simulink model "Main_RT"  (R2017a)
settings: Solver=VariableStepAuto  StartTime=0.0  StopTime=50  FixedStep=1  RelTol=1e-3
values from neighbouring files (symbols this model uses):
  Hs_swlRange = zeros(states,N)    [run_master.m]
  Hsd_seaRange = zeros(states,N)    [run_master.m]
  Hsd_swlRange = zeros(states,N)    [run_master.m]
  m = 0    [wavespec.m]
  MC_Hs_swl = zeros(states,states,N)    [run_master.m]
  MC_Hsd_sea = zeros(states,states,N)    [run_master.m]
  MC_Hsd_swl = zeros(states,states,N)    [run_master.m]
  MC_Tp_sea = zeros(states,states,N)    [run_master.m]
  MC_Tp_swl = zeros(states,states,N)    [run_master.m]
  MC_u10 = zeros(states,states,N)    [run_master.m]
  MC_u10d = zeros(states,states,N)    [run_master.m]
  n = 0    [wavespec.m]
  Random_Values = generate_random_matrix(seed,SetNumRTs)    [run_master.m]    (also in generate_random_matrix.m = rand(Num_rand,8))
  Tp_seaRange = zeros(states,N)    [run_master.m]
  Tp_swlRange = zeros(states,N)    [run_master.m]
  u10_Range = zeros(states,N)    [run_master.m]
  u10d_Range = zeros(states,N)    [run_master.m]
  v_req_start = 14.5    [run_master.m]
  wpts = [32.8502 121.2880    [run_master.m]
undefined symbols (not defined in the file or in its folder): course_legs, course_legsBA, distnm_legs, distnm_legsBA, Hs_seaRange, MC_Hs_sea, ship_cargo_capacity

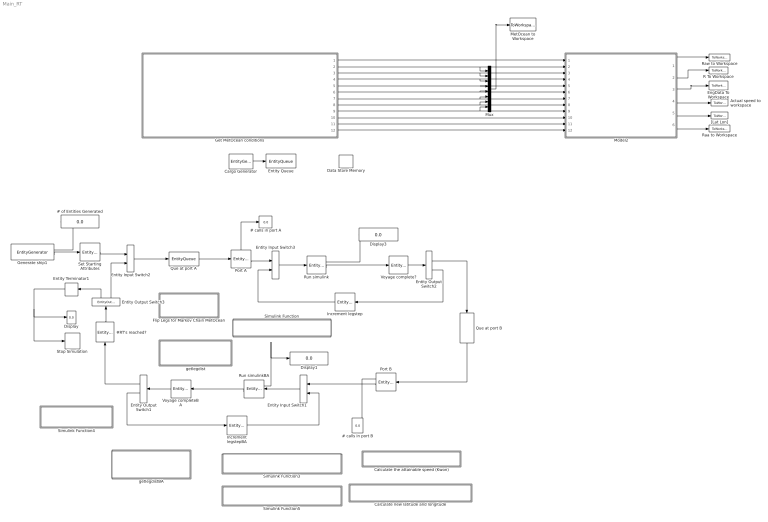
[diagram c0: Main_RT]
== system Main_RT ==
  # calls in port A : Display
  # calls in port B : Display
  # of Entities Generated : Display
  #RT's reached? : EntityServer  InputPortMessageModes=m  OutputPortMessageModes=m  Capacity=1  ServiceTimeValue=0  EntryAction=|
      | %Add to the number of round trips (RTs) completed
      | entity.NumRTs=entity.NumRTs+1;
      | 
      | %Check to see if the desired number of RTs is reached
      | %If so, send entity to terminate simulation
      | entity.outputport=Completed_RT(entity.NumRTs);
  Actual speed to workspace : ToWorkspace  VariableName=V_act  SaveFormat=Timeseries  SampleTime=-1
  Calculate new latitude and longitude : Subsystem  TreatAsAtomicUnit=on
  Calculate the attainable speed (Kwon) : Subsystem  TreatAsAtomicUnit=on
  Cargo Generator : EntityGenerator  Commented=on  OutputPortMessageModes=m  EntityType=Structured  EntityTypeName=Entity
  Data Store Memory : DataStoreMemory  ReadBeforeWriteMsg=warning  WriteAfterWriteMsg=warning  WriteAfterReadMsg=warning  ShowAdditionalParam=off
  Display : Display
  Display1 : Display
  Display3 : Display
  EngData To Workspace : ToWorkspace  VariableName=engroom  SaveFormat=Timeseries  SampleTime=-1
  Entity Input Switch1 : EntityInputSwitch  InputPortMessageModes=m,m  OutputPortMessageModes=m
  Entity Input Switch2 : EntityInputSwitch  InputPortMessageModes=m,m  OutputPortMessageModes=m
  Entity Input Switch3 : EntityInputSwitch  InputPortMessageModes=m,m  OutputPortMessageModes=m
  Entity Output Switch1 : EntityOutputSwitch  InputPortMessageModes=m  OutputPortMessageModes=m,m  SwitchingCriterion=From attribute  SwitchAttributeName=outputport
  Entity Output Switch2 : EntityOutputSwitch  InputPortMessageModes=m  OutputPortMessageModes=m,m  SwitchingCriterion=From attribute  SwitchAttributeName=outputport
  Entity Output Switch3 : EntityOutputSwitch  InputPortMessageModes=m  OutputPortMessageModes=m,m  SwitchingCriterion=From attribute  SwitchAttributeName=outputport
  Entity Queue : EntityQueue  Commented=on  InputPortMessageModes=m  OutputPortMessageModes=m
  Entity Terminator1 : EntityTerminator  InputPortMessageModes=m  NumberEntitiesArrived=on
  Flip Legs for Markov Chain MetOcean : Subsystem  TreatAsAtomicUnit=on
  Generate ship1 : EntityGenerator  OutputPortMessageModes=n,m  TimeSource=MATLAB action  IntergenerationTimeAction=|  GenerateEntityAtSimulationStart=off  AttributeName=HsSea_S|HsdSea_S|TpSea_S|HsSwl_S|HsdSwl_S|TpSwl_S|u10_S|u10d_S|speed|outputport|legstep|legdist|leg|course|lat|lon|Hs4k|Hsd4k|Att_speed|Dist_sailed_tot|Dist_sailed_leg|NumRTs|Voyage_step|capacity  AttributeInitialValue=0|0|0|0|0|0|0|0|15|1|2|1|1|1|1|1|1|1|1|0|0|0|0|1  NumberEntitiesDeparted=on  EntityType=Structured  EntityTypeName=ship
      | persistent count igt;
      | if isempty(count)
      |     igt=[0 inf];
      |     count=1;
      | end
      | dt=igt(count);
      | count=count+1;
  Get MetOcean conditions : Subsystem  TreatAsAtomicUnit=on
  Increment legstep : EntityServer  InputPortMessageModes=m  OutputPortMessageModes=m  Capacity=1  ServiceTimeValue=0  EntryAction=|
      | %increment the total progress
      | entity.legstep=entity.legstep+1;
  Increment legstepBA : EntityServer  InputPortMessageModes=m  OutputPortMessageModes=m  Capacity=1  ServiceTimeValue=0  EntryAction=|
      | %increment the total progress
      | entity.legstep=entity.legstep+1;
  MetOcean to Workspace : ToWorkspace  VariableName=MetOcean  SaveFormat=Timeseries  SampleTime=-1
  Model2 : ModelReference  ModelNameDialog=Ship_Model  SimulationMode=Normal  ModelReferenceVersion=1.112
  Mux : Mux  Inputs=8
  Port A : EntityServer  InputPortMessageModes=m  OutputPortMessageModes=n,m  Capacity=1  ServiceTimeValue=10  EntryAction=|  NumberEntitiesDeparted=on
      | %The ship is in port
      | 
      | %Run the ship model with the following modifications
      | %speed=0
      | %course=0
      | %Voyage_step: +0.5 (read as vessel being in port)
      | 
      | %run the ship model  and output the weather states (Markov Chain)
      | [HsSea_S,HsdSea_S,TpSea_S,HsSwl_S,HsdSwl_S,TpSwl_S,hsd4k,hs4k,u10_S,u10d_S]=runSim(entity.legstep, entity.course,entity.speed,entity.leg,...
      |                                                 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
  Port B : EntityServer  InputPortMessageModes=m  OutputPortMessageModes=n,m  Capacity=1  ServiceTimeValue=10  EntryAction=|  NumberEntitiesDeparted=on
      | %The ship is in port
      | 
      | %Run the ship model with the following modifications
      | %speed=0
      | %course=0
      | %Voyage_step: +0.5 (read as vessel being in port)
      | 
      | %run the ship model  and output the weather states (Markov Chain)
      | [HsSea_S,HsdSea_S,TpSea_S,HsSwl_S,HsdSwl_S,TpSwl_S,hsd4k,hs4k,u10_S,u10d_S]=runSim(entity.legstep, 0,0,entity.leg,...
      |                                                            entity.HsSwl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
  Que at port A : EntityQueue  InputPortMessageModes=m  OutputPortMessageModes=m
  Que at port B : EntityQueue  InputPortMessageModes=m  OutputPortMessageModes=m
  R To Workspace : ToWorkspace  VariableName=R  SaveFormat=Timeseries  SampleTime=-1
  Raa to Workspace : ToWorkspace  VariableName=Raa  SaveFormat=Timeseries  SampleTime=-1
  Raw to Workspace : ToWorkspace  VariableName=Raw  SaveFormat=Timeseries  SampleTime=-1
  Run simulink : EntityServer  InputPortMessageModes=m  OutputPortMessageModes=n,m  Capacity=1  ServiceTimeValue=1  EntryAction=|  NumberEntitiesDeparted=on
      | %take the current leg, and give the vessel its course and the distance of the leg
      | [entity.course,entity.legdist]=readLeg(entity.leg);
      | 
      | %run the ship model, and output the weather states (Markov Chain)
      | [HsSea_S,HsdSea_S,TpSea_S,HsSwl_S,HsdSwl_S,...
      |         TpSwl_S,hsd4k,hs4k,u10_S,u10d_S]  =  runSim(entity.legstep, entity.course,entity.speed,entity.leg,...
      |                                           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
  Run simulinkBA : EntityServer  InputPortMessageModes=m  OutputPortMessageModes=n,m  Capacity=1  ServiceTimeValue=1  EntryAction=|  NumberEntitiesDeparted=on
      | %take the current leg, and give the vessel its course and the distance of the leg
      | [entity.course,entity.legdist]=readLegBA(entity.leg); %reads from the flipped waypoints
      | 
      | %Flip leg number to collect the correct weather data for Markov Chain MetOcean
      | mc_leg=getmcleg(entity.leg);
      | 
      | %run the ship model, and output the weather states (Markov Chain)
      | [HsSea_S,HsdSea_S,TpSea_S,HsSwl_S,HsdSwl_S,...
      |        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
  Set Starting Attributes : EntityServer  InputPortMessageModes=m  OutputPortMessageModes=m  Capacity=1  ServiceTimeValue=0  EntryAction=|
      | %Read origin coordinates from waypoints
      | [lat1,lon1,v_req,capacity]=SetStart();
      | 
      | %Assign starting coordinates to entity
      | entity.lat=lat1;
      | entity.lon=lon1;
      | 
      | %Assign the intended speed
      | entity.speed=v_req;
      | 
      | %Assign cargo capacity
      | entity.capacity=capacity;
  Simulink Function : Subsystem  TreatAsAtomicUnit=on
  Simulink Function3 : Subsystem  TreatAsAtomicUnit=on
  Simulink Function4 : Subsystem  TreatAsAtomicUnit=on
  Simulink Function5 : Subsystem  TreatAsAtomicUnit=on
  Stop Simulation : Stop
  Voyage complete? : EntityServer  InputPortMessageModes=m  OutputPortMessageModes=m  Capacity=1  ServiceTimeValue=0  EntryAction=entity.outputport=checkComplete(entity.leg,entity.legdist,entity.Dist_sailed_leg);
  Voyage completeBA : EntityServer  InputPortMessageModes=m  OutputPortMessageModes=m  Capacity=1  ServiceTimeValue=0  EntryAction=entity.outputport=checkCompleteBA(entity.leg,entity.legdist,entity.Dist_sailed_leg);
  "[Lat Lon]" : ToWorkspace  VariableName=LatLon  SaveFormat=Timeseries  SampleTime=-1
  getlegdist : Subsystem  TreatAsAtomicUnit=on
  getlegdistBA : Subsystem  TreatAsAtomicUnit=on
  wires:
  Que at port B/1 -> Port B/1
  Entity Output Switch1/2 -> Increment legstepBA/1
  Port B/2 -> Entity Input Switch1/1
  Entity Input Switch1/1 -> Run simulinkBA/1
  Entity Input Switch2/1 -> Que at port A/1
  Cargo Generator/1 -> Entity Queue/1
  Model2/4 -> Actual speed to workspace/1
  Model2/2 -> R To Workspace/1
  Get MetOcean conditions/3(relD_sea) -> Model2/3, Mux/2
  Get MetOcean conditions/5(Hs_swl) -> Mux/4, Model2/5
  Get MetOcean conditions/2(Hs_sea) -> Mux/1, Model2/2
  Get MetOcean conditions/7(Tp_swl) -> Mux/6, Model2/7
  Get MetOcean conditions/1(vreq) -> Model2/1
  Model2/5 -> "[Lat Lon]"/1
  Model2/1 -> Raw to Workspace/1
  Get MetOcean conditions/6(relD_swl) -> Mux/5, Model2/6
  Get MetOcean conditions/4(Tp_sea) -> Mux/3, Model2/4
  Mux/1 -> MetOcean to Workspace/1
  Model2/3 -> EngData To Workspace/1
  Generate ship1/2 -> Set Starting Attributes/1
  Set Starting Attributes/1 -> Entity Input Switch2/1
  Generate ship1/1 -> # of Entities Generated/1
  Run simulinkBA/2 -> Voyage completeBA/1
  Voyage completeBA/1 -> Entity Output Switch1/1
  Increment legstepBA/1 -> Entity Input Switch1/2
  Run simulinkBA/1 -> Display1/1
  Port A/1 -> # calls in port A/1
  Port B/1 -> # calls in port B/1
  Entity Terminator1/1 -> Stop Simulation/1, Display/1
  Entity Output Switch3/2 -> Entity Input Switch2/2
  Entity Output Switch3/1 -> Entity Terminator1/1
  #RT's reached?/1 -> Entity Output Switch3/1
  Entity Output Switch1/1 -> #RT's reached?/1
  Entity Output Switch2/1 -> Que at port B/1
  Run simulink/1 -> Display3/1
  Entity Output Switch2/2 -> Increment legstep/1
  Voyage complete?/1 -> Entity Output Switch2/1
  Run simulink/2 -> Voyage complete?/1
  Increment legstep/1 -> Entity Input Switch3/2
  Entity Input Switch3/1 -> Run simulink/1
  Port A/2 -> Entity Input Switch3/1
  Que at port A/1 -> Port A/1
  Get MetOcean conditions/8(u10) -> Model2/8, Mux/7
  Get MetOcean conditions/9(relD_u10) -> Model2/9, Mux/8
  Get MetOcean conditions/10(Course) -> Model2/10
  Get MetOcean conditions/11(lat) -> Model2/11
  Get MetOcean conditions/12(lon) -> Model2/12
  Model2/6 -> Raa to Workspace/1

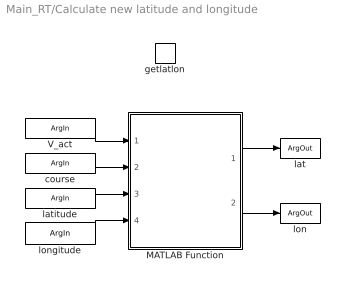
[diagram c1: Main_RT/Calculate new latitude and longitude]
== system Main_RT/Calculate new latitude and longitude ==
  getlatlon : TriggerPort  TriggerType=function-call  IsSimulinkFunction=on  FunctionName=getlatlon  VariantControl=Variant
  MATLAB Function : MATLAB Function  TreatAsAtomicUnit=on
  V_act : ArgIn  DisableCoverage=on  ArgumentName=V_act
  latitude : ArgIn  Port=2  ArgumentName=latitude
  longitude : ArgIn  Port=3  ArgumentName=longitude
  course : ArgIn  Port=4  ArgumentName=course
  lat : ArgOut  DisableCoverage=on  ArgumentName=lat
  lon : ArgOut  Port=2  ArgumentName=lon
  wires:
  V_act/1 -> MATLAB Function/1(V_act)
  MATLAB Function/1(lat_new) -> lat/1
  course/1 -> MATLAB Function/2(Course)
  latitude/1 -> MATLAB Function/3(Lat)
  longitude/1 -> MATLAB Function/4(Lon)
  MATLAB Function/2(lon_new) -> lon/1

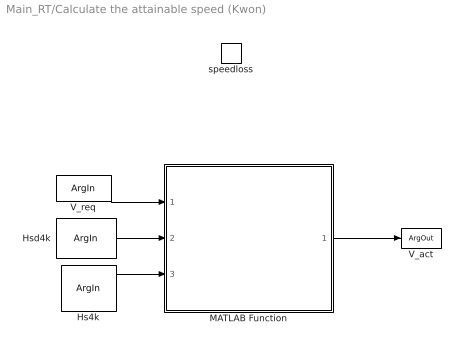
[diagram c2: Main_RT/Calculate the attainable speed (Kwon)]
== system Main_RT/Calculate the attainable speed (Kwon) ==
  speedloss : TriggerPort  TriggerType=function-call  IsSimulinkFunction=on  FunctionName=speedloss  VariantControl=Variant
  MATLAB Function : MATLAB Function  TreatAsAtomicUnit=on
  V_req : ArgIn  DisableCoverage=on  ArgumentName=V_req
  Hsd4k : ArgIn  Port=2  ArgumentName=Hsd4k
  Hs4k : ArgIn  Port=3  ArgumentName=Hs4k
  V_act : ArgOut  DisableCoverage=on  ArgumentName=V_act
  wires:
  MATLAB Function/1(V_act) -> V_act/1
  Hs4k/1 -> MATLAB Function/3(Hs)
  Hsd4k/1 -> MATLAB Function/2(rel_heading)
  V_req/1 -> MATLAB Function/1(V_req)

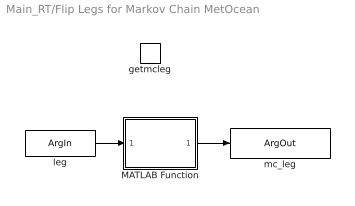
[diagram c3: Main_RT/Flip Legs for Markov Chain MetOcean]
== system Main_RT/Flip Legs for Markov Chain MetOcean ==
  getmcleg : TriggerPort  TriggerType=function-call  IsSimulinkFunction=on  FunctionName=getmcleg  VariantControl=Variant
  MATLAB Function : MATLAB Function  TreatAsAtomicUnit=on
  leg : ArgIn  DisableCoverage=on  ArgumentName=leg
  mc_leg : ArgOut  DisableCoverage=on  ArgumentName=mc_leg
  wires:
  leg/1 -> MATLAB Function/1(leg)
  MATLAB Function/1(mc_leg) -> mc_leg/1

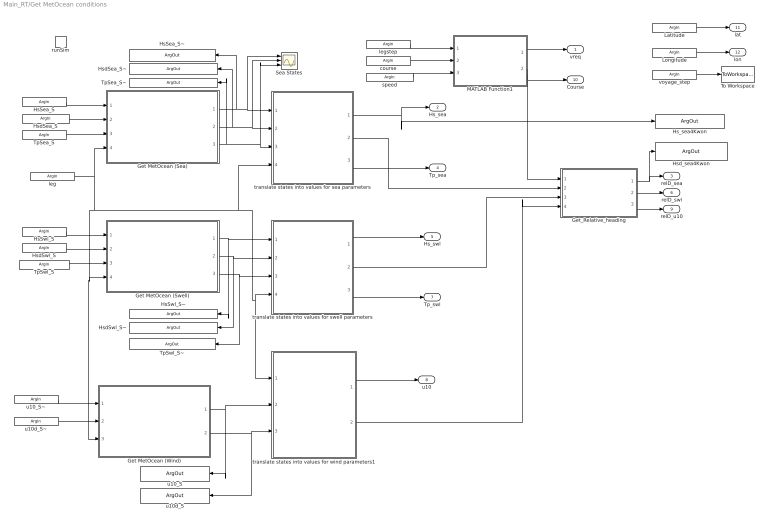
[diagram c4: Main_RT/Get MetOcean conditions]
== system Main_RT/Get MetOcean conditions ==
  runSim : TriggerPort  TriggerType=function-call  IsSimulinkFunction=on  FunctionName=runSim  VariantControl=Variant
  Get MetOcean (Sea) : MATLAB Function  TreatAsAtomicUnit=on
  Get MetOcean (Swell) : MATLAB Function  TreatAsAtomicUnit=on
  Get MetOcean (Wind) : MATLAB Function  TreatAsAtomicUnit=on
  Get_Relative_heading : MATLAB Function  TreatAsAtomicUnit=on
  MATLAB Function1 : MATLAB Function  TreatAsAtomicUnit=on
  Sea States : Scope  NumInputPorts=3
  To Workspace : ToWorkspace  VariableName=voyage_step  SaveFormat=Timeseries  SampleTime=-1
  translate states into values for swell parameters : MATLAB Function  TreatAsAtomicUnit=on
  translate states into values for wind parameters1 : MATLAB Function  TreatAsAtomicUnit=on
  translate states into values for sea parameters : MATLAB Function  TreatAsAtomicUnit=on
  legstep : ArgIn  ArgumentName=legstep
  course : ArgIn  Port=2  ArgumentName=course
  speed : ArgIn  Port=3  ArgumentName=speed
  leg : ArgIn  Port=4  ArgumentName=leg
  HsSwl_S : ArgIn  Port=5  ArgumentName=HsSwl_S
  HsdSwl_S : ArgIn  Port=6  ArgumentName=HsdSwl_S
  TpSwl_S : ArgIn  Port=7  ArgumentName=TpSwl_S
  HsSea_S : ArgIn  Port=8  ArgumentName=HsSea_S
  HsdSea_S : ArgIn  Port=9  ArgumentName=HsdSea_S
  TpSea_S : ArgIn  Port=10  ArgumentName=TpSea_S
  Latitude : ArgIn  Port=11  ArgumentName=Latitude
  Longitude : ArgIn  Port=12  ArgumentName=Longitude
  u10_S~ : ArgIn  Port=13  ArgumentName=u10_S
  u10d_S~ : ArgIn  Port=14  ArgumentName=u10d_S
  voyage_step : ArgIn  Port=15  ArgumentName=voyage_step
  HsSea_S~ : ArgOut  ArgumentName=HsSea_S
  HsdSea_S~ : ArgOut  Port=2  ArgumentName=HsdSea_S
  TpSea_S~ : ArgOut  Port=3  ArgumentName=TpSea_S
  HsSwl_S~ : ArgOut  Port=4  ArgumentName=HsSwl_S
  HsdSwl_S~ : ArgOut  Port=5  ArgumentName=HsdSwl_S
  TpSwl_S~ : ArgOut  Port=6  ArgumentName=TpSwl_S
  Hsd_sea4Kwon : ArgOut  Port=7  ArgumentName=Hsd_sea4Kwon
  Hs_sea4Kwon : ArgOut  Port=8  ArgumentName=Hs_sea4Kwon
  u10_S : ArgOut  Port=9  ArgumentName=u10_S
  u10d_S : ArgOut  Port=10  ArgumentName=u10d_S
  vreq : Outport
  Hs_sea : Outport  Port=2
  relD_sea : Outport  Port=3
  Tp_sea : Outport  Port=4
  Hs_swl : Outport  Port=5
  relD_swl : Outport  Port=6
  Tp_swl : Outport  Port=7
  u10 : Outport  Port=8
  relD_u10 : Outport  Port=9
  Course : Outport  Port=10
  lat : Outport  Port=11
  lon : Outport  Port=12
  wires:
  leg/1 -> Get MetOcean (Sea)/4(leg), Get MetOcean (Wind)/3(leg), Get MetOcean (Swell)/4(leg), translate states into values for wind parameters1/1(leg), translate states into values for swell parameters/4(leg), translate states into values for sea parameters/4(leg)
  Get MetOcean (Sea)/1(Sea_HSS) -> HsSea_S~/1, Sea States/1, translate states into values for sea parameters/1(HsSea_S)
  Get MetOcean (Sea)/2(Sea_HSDS) -> HsdSea_S~/1, Sea States/2, translate states into values for sea parameters/2(HsdSea_S)
  Get MetOcean (Sea)/3(Sea_TPS) -> TpSea_S~/1, Sea States/3, translate states into values for sea parameters/3(TpSea_S)
  translate states into values for sea parameters/1(Hs_sea) -> Hs_sea4Kwon/1, Hs_sea/1
  translate states into values for sea parameters/3(Tp_sea) -> Tp_sea/1
  Get MetOcean (Swell)/2(HSD_S) -> HsdSwl_S~/1, translate states into values for swell parameters/2(HsdSwl_S)
  Get MetOcean (Swell)/3(TM_S) -> TpSwl_S~/1, translate states into values for swell parameters/3(TpSwl_S)
  translate states into values for swell parameters/2(Hsd_swl) -> Get_Relative_heading/3(Hsd_swl)
  Get MetOcean (Swell)/1(HS_S) -> HsSwl_S~/1, translate states into values for swell parameters/1(HsSwl_S)
  translate states into values for swell parameters/1(Hs_swl) -> Hs_swl/1
  translate states into values for swell parameters/3(Tp_swl) -> Tp_swl/1
  MATLAB Function1/1(Vreq) -> vreq/1
  MATLAB Function1/2(Course) -> Get_Relative_heading/1(course), Course/1
  HsSea_S/1 -> Get MetOcean (Sea)/1(Hs_SeS)
  HsdSea_S/1 -> Get MetOcean (Sea)/2(Hsd_SeS)
  TpSea_S/1 -> Get MetOcean (Sea)/3(Tp_SeS)
  TpSwl_S/1 -> Get MetOcean (Swell)/3(Per_S)
  HsdSwl_S/1 -> Get MetOcean (Swell)/2(Head_S)
  HsSwl_S/1 -> Get MetOcean (Swell)/1(Wave_S)
  speed/1 -> MATLAB Function1/3(speed)
  course/1 -> MATLAB Function1/2(course)
  legstep/1 -> MATLAB Function1/1(legstep)
  Latitude/1 -> lat/1
  Longitude/1 -> lon/1
  u10_S~/1 -> Get MetOcean (Wind)/1(windVel_S)
  translate states into values for wind parameters1/1(u10) -> u10/1
  translate states into values for sea parameters/2(Hsd_sea) -> Get_Relative_heading/2(Hsd_sea)
  translate states into values for wind parameters1/2(u10d) -> Get_Relative_heading/4(u10d)
  Get_Relative_heading/3(relD_u10) -> relD_u10/1
  Get_Relative_heading/2(relD_swl) -> relD_swl/1
  Get_Relative_heading/1(relD_sea) -> Hsd_sea4Kwon/1, relD_sea/1
  Get MetOcean (Wind)/1(u10_S) -> u10_S/1, translate states into values for wind parameters1/2(u10_S)
  Get MetOcean (Wind)/2(u10d_S) -> u10d_S/1, translate states into values for wind parameters1/3(u10d_S)
  u10d_S~/1 -> Get MetOcean (Wind)/2(windDir_S)
  voyage_step/1 -> To Workspace/1

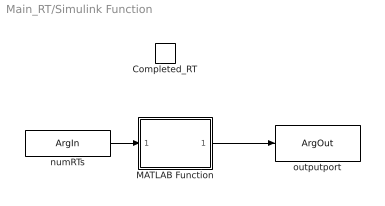
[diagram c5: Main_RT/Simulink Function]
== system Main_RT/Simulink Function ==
  Completed_RT : TriggerPort  TriggerType=function-call  IsSimulinkFunction=on  FunctionName=Completed_RT  VariantControl=Variant
  MATLAB Function : MATLAB Function  TreatAsAtomicUnit=on
  numRTs : ArgIn  DisableCoverage=on  ArgumentName=numRTs
  outputport : ArgOut  DisableCoverage=on  ArgumentName=outputport
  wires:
  numRTs/1 -> MATLAB Function/1(NumRTs)
  MATLAB Function/1(outport) -> outputport/1

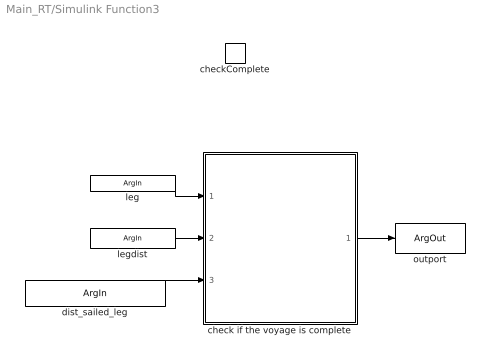
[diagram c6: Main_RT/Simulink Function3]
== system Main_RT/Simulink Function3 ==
  checkComplete : TriggerPort  TriggerType=function-call  IsSimulinkFunction=on  FunctionName=checkComplete  VariantControl=Variant
  check if the voyage is complete : MATLAB Function  TreatAsAtomicUnit=on
  leg : ArgIn  DisableCoverage=on  ArgumentName=leg
  legdist : ArgIn  Port=2  ArgumentName=legdist
  dist_sailed_leg : ArgIn  Port=3  ArgumentName=dist_sailed_leg
  outport : ArgOut  DisableCoverage=on  ArgumentName=outport
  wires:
  leg/1 -> check if the voyage is complete/1(leg)
  check if the voyage is complete/1(outport) -> outport/1
  dist_sailed_leg/1 -> check if the voyage is complete/3(dist_sailed_leg)
  legdist/1 -> check if the voyage is complete/2(legdist)

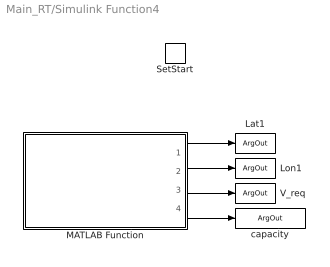
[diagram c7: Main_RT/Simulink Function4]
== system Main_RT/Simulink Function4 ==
  SetStart : TriggerPort  TriggerType=function-call  IsSimulinkFunction=on  FunctionName=SetStart  VariantControl=Variant
  MATLAB Function : MATLAB Function  TreatAsAtomicUnit=on
  Lat1 : ArgOut  DisableCoverage=on  ArgumentName=Lat1
  Lon1 : ArgOut  Port=2  ArgumentName=Lon1
  V_req : ArgOut  Port=3  ArgumentName=V_req
  capacity : ArgOut  Port=4  ArgumentName=capacity
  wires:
  MATLAB Function/2(Lon1) -> Lon1/1
  MATLAB Function/1(Lat1) -> Lat1/1
  MATLAB Function/3(v_req) -> V_req/1
  MATLAB Function/4(capacity) -> capacity/1

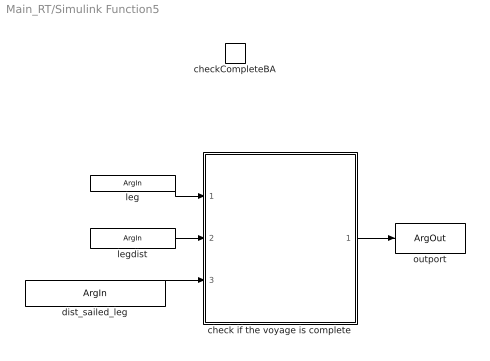
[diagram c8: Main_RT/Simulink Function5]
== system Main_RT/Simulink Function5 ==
  checkCompleteBA : TriggerPort  TriggerType=function-call  IsSimulinkFunction=on  FunctionName=checkCompleteBA  VariantControl=Variant
  check if the voyage is complete : MATLAB Function  TreatAsAtomicUnit=on
  leg : ArgIn  DisableCoverage=on  ArgumentName=leg
  legdist : ArgIn  Port=2  ArgumentName=legdist
  dist_sailed_leg : ArgIn  Port=3  ArgumentName=dist_sailed_leg
  outport : ArgOut  DisableCoverage=on  ArgumentName=outport
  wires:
  leg/1 -> check if the voyage is complete/1(leg)
  check if the voyage is complete/1(outport) -> outport/1
  dist_sailed_leg/1 -> check if the voyage is complete/3(dist_sailed_leg)
  legdist/1 -> check if the voyage is complete/2(legdist)

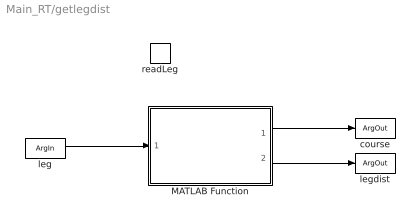
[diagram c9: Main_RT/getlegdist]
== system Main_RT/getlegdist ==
  readLeg : TriggerPort  TriggerType=function-call  IsSimulinkFunction=on  FunctionName=readLeg  VariantControl=Variant
  MATLAB Function : MATLAB Function  TreatAsAtomicUnit=on
  leg : ArgIn  DisableCoverage=on  ArgumentName=leg
  course : ArgOut  DisableCoverage=on  ArgumentName=course
  legdist : ArgOut  DisableCoverage=on  Port=2  ArgumentName=legdist
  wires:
  leg/1 -> MATLAB Function/1(leg)
  MATLAB Function/1(course) -> course/1
  MATLAB Function/2(legdist) -> legdist/1

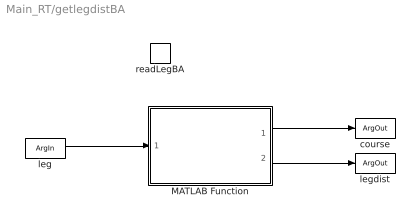
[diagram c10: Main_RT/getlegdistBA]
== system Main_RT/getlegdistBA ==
  readLegBA : TriggerPort  TriggerType=function-call  IsSimulinkFunction=on  FunctionName=readLegBA  VariantControl=Variant
  MATLAB Function : MATLAB Function  TreatAsAtomicUnit=on
  leg : ArgIn  DisableCoverage=on  ArgumentName=leg
  course : ArgOut  DisableCoverage=on  ArgumentName=course
  legdist : ArgOut  DisableCoverage=on  Port=2  ArgumentName=legdist
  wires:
  leg/1 -> MATLAB Function/1(leg)
  MATLAB Function/1(course) -> course/1
  MATLAB Function/2(legdist) -> legdist/1

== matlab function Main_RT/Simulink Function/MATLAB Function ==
function outport = outputportRT(NumRTs,SetNumRTs)



if NumRTs>=SetNumRTs
outport = 1; %Simulation is complete, end simulation
else
    outport=2; %Simulation is not complete, do another roundtrip
end
end

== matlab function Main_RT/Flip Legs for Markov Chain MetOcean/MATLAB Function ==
function mc_leg = getMCleg(leg,distnm_legsBA)

%Flip the leg number to collect the correct weather data for MetOcean
%Markov Chains

num_legs=size(distnm_legsBA,1); %get the total number of legs
legs=(1:1:num_legs);
flip_legs=flip(legs);
mc_leg=flip_legs(leg);
end

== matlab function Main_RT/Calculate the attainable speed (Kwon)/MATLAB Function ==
function V_act = speedloss_Kwon(V_req,rel_heading,Hs, num)
coder.extrinsic('wrapTo180')
%Use Kwons method to estimate the speed loss due to added resistance

%pre allocate values
V_act=0;
V_2=0; %pre allocate the new speed
Bn=0;
Volume_deplacement=0;
C_u=0;
C_beta=0;
C_form=0;
heading_rel=0;

V_1=V_req*0.5144; %Convert the required speed (set speed) from kts to m/s
heading_rel=abs(wrapTo180(rel_heading)); %convert to 0-180 degrees
Volume_deplacement=num(54); %[m^3]
L=num(3); %Use Lwl
C_B=num(8); %block Coefficient



%calculate the current Froude Number
F_n=V_1/((9.81*L)^0.5);

%Get Beaufort scale number from waveheight
if Hs<0.2
    Bn=1;
elseif Hs>=0.2 && Hs<0.5
    Bn=2;
elseif Hs>=0.5 && Hs<1
    Bn=3;
elseif Hs>=1 && Hs<2
    Bn=4;
elseif Hs>2 && Hs<3
    Bn=5;
elseif Hs>3 && Hs<4
    Bn=6;
elseif Hs>4 %&& Hs<5.5
    Bn=7;
else
    disp('Bn is too high for Kwons method')
end
    

%calculate speed reduction coefficient
if C_B>=0.55 && C_B<0.575
    C_u=1.7-(1.4*F_n)-(7.4*(F_n^2));
elseif C_B>=0.575 && C_B<0.625
    C_u=2.2-(2.5*F_n)-(9.7*(F_n^2));
elseif C_B>=0.625 && C_B<0.675
    C_u=2.6-(3.7*F_n)-(11.6*(F_n^2));
elseif C_B>=0.675 && C_B<0.725
    C_u=3.1-(5.3*F_n)-(12.4*(F_n^2));
elseif C_B>=0.725 && C_B<0.775
    C_u=2.4-(10.6*F_n)-(9.5*(F_n^2));
elseif C_B>=0.775 && C_B<0.825
    C_u=2.6-(13.1*F_n)-(15.1*(F_n^2));
else %C_B>=0.825
    C_u=3.1-(18.7*F_n)+(28*(F_n^2));
end

%calculate direction reduction coefficient
if heading_rel>=0 && heading_rel<30 %head sea
    C_beta=1;
elseif heading_rel>=30 && heading_rel<60 %Bow sea
    C_beta=(1.7-0.03*((Bn-4)^2))/2;
elseif heading_rel>=60 && heading_rel<150 %Beam sea
    C_beta=(0.9-0.06*((Bn-6)^2))/2;
else %heading_rel>=150 && heading_rel<180 %Following sea
    C_beta=(0.4-0.03*((Bn-8)^2))/2;
end

%calculate the ship form coefficient
%valid for all ships, exept container ships, in loaded condition
%C_form=(0.5*Bn)+((Bn^(6.5))/((2.7*(Volume_deplacement^(2/3)))));

%valid for container ships in normal condition
C_form=(0.7*Bn)+((Bn^(6.5))/((22*(Volume_deplacement^(2/3)))));

%percentage loss calculated
%percentage_loss=((V_1-V_2)/V_1)*100;





%calculate deltaV/V1*100%
%Delta_V_overV=C_beta*C_u*C_form;
%coefficient=C_form*C_beta*C_u
%calculate actual ship speed in the selected weather [m/s]
% V_2=V_1-((Delta_V_overV)*(V_1/100))
V_2=V_1-((C_beta*C_u*C_form)*(V_1/100));

%calculate the absolute speed loss [m/s]
%delta_V=V_1-V_2



%if the speed loss found is negative, set the speed to the original speed
% This means that the approximate method did not work in this case
% if V_2>=V_1
%     V_2=V_1; 
%     disp('Approximate method not valid')
%     
% end

V_act=V_2/0.5144; % The actual attainable speed in kts
end


% %function V_act = speedloss_Kwon(V_req,rel_heading,Hs, num)
% %Use Kwons method to estimate the speed loss due to added resistance
% 
% V_1=V_req*0.5144; %Convert the required speed (set speed) from kts to m/s
% heading_rel=rel_heading;
% Volume_deplacement=num(54); %[m^3]
% L=num(3); %Use Lwl
% C_B=num(8); %block Coefficient
% 
% 
% %calculate the current Froude Number
% F_n=V_1/((9.81*L)^0.5);
% 
% %Get Beaufort scale number from waveheight
% if Hs<0.2
%     Bn=1;
% elseif Hs>=0.2 && Hs<0.5
%     Bn=2;
% elseif Hs>=0.5 && Hs<1
%     Bn=3;
% elseif Hs>=1 && Hs<2
%     Bn=4;
% elseif Hs>2 && Hs<3
%     Bn=5;
% elseif Hs>3 && Hs<4
%     Bn=6;
% elseif Hs>4 && Hs<5.5
%     Bn=7;
% else
%     disp('Bn is too high for Kwons method')
% end
%     
% 
% %calculate speed reduction coefficient
% if C_B>=0.55 && C_B<0.575
%     C_u=1.7-(1.4*F_n)-(7.4*(F_n^2));
% elseif C_B>=0.575 && C_B<0.625
%     C_u=2.2-(2.5*F_n)-(9.7*(F_n^2));
% elseif C_B>=0.625 && C_B<0.675
%     C_u=2.6-(3.7*F_n)-(11.6*(F_n^2));
% elseif C_B>=0.675 && C_B<0.725
%     C_u=3.1-(5.3*F_n)-(12.4*(F_n^2));
% elseif C_B>=0.725 && C_B<0.775
%     C_u=2.4-(10.6*F_n)-(9.5*(F_n^2));
% elseif C_B>=0.775 && C_B<0.825
%     C_u=2.6-(13.1*F_n)-(15.1*(F_n^2));
% elseif C_B>=0.825
%     C_u=3.1-(18.7*F_n)+(28*(F_n^2));
% end
% 
% %calculate direction reduction coefficient
% if heading_rel>=0 && heading_rel<30 %head sea
%     C_beta=1;
% elseif heading_rel>=30 && heading_rel<60 %Bow sea
%     C_beta=(1.7-0.03*((Bn-4)^2))/2;
% elseif heading_rel>=60 && heading_rel<150 %Beam sea
%     C_beta=(0.9-0.06*((Bn-6)^2))/2;
% elseif heading_rel>=150 && heading_rel<180 %Following sea
%     C_beta=(0.4-0.03*((Bn-8)^2))/2;
% end
% 
% %calculate the ship form coefficient
% %valid for all ships, exept container ships, in loaded condition
% C_form=(0.5*Bn)+((Bn^(6.5))/((2.7*(Volume_deplacement^(2/3)))));
% 
% %calculate deltaV/V1*100%
% %Delta_V_overV=C_beta*C_u*C_form;
% 
% %calculate actual ship speed in the selected weather [m/s]
% % V_2=V_1-((Delta_V_overV)*(V_1/100))
% V_2=V_1-((C_beta*C_u*C_form)*(V_1/100));
% 
% %calculate the absolute speed loss [m/s]
% %delta_V=V_1-V_2
% 
% %percentage loss calculated
% %percentage_loss=((V_1-V_2)/V_1)*100;
% 
% %if the speed loss found is negative, set the speed to the original speed
% % This means that the approximate method did not work in this case
% if V_2>=V_1
%     V_2=V_1; 
%     disp('Approximate method not valid')
%     
% end
% 
% V_act=V_2/0.5144; % The actual attainable speed in kts
% 
% end

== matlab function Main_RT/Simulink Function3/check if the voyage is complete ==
function outport = fcn(leg,legdist,dist_sailed_leg,distnm_legs)

dist=dist_sailed_leg; %the distance sailed on current leg

if leg == length(distnm_legs) && dist>=(legdist-20) %subtract to avoid errors
    outport=1; %Journey complete
else
    outport=2; %Journey not complete
end

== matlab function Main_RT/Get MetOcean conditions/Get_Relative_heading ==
function [relD_sea, relD_swl, relD_u10] = fcn(course, Hsd_sea, Hsd_swl, u10d)

relD_sea = (Hsd_sea-course);
relD_swl = (Hsd_swl-course);
relD_u10 = (u10d-course);

end

== matlab function Main_RT/Get MetOcean conditions/translate states into values
for swell parameters ==
function [Hs_swl, Hsd_swl, Tp_swl] = weatherValues(HsSwl_S, HsdSwl_S, TpSwl_S, leg, Hs_swlRange, Hsd_swlRange, Tp_swlRange)

Hs_swl = Hs_swlRange(HsSwl_S, leg);
Hsd_swl = Hsd_swlRange(HsdSwl_S, leg);
Tp_swl = Tp_swlRange(TpSwl_S, leg);

end

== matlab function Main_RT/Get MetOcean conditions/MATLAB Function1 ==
function [Vreq, Course]  = fcn(legstep, course, speed)



%pre-allocating as integers to avoid error message
% heading=0;
% period=0;
% Hs=0;

%declare these functions as extrinsic to be able to use them in simulink
%block
% coder.extrinsic('sprintf');
% coder.extrinsic('xlsread');

%If location has changed, then we can change what spreadsheet we look at,
%but for now we use the same spreadsheet

% filename = 'weatherinput.xlsx';
% xlRange = sprintf('B%d:BB%d',legstep,legstep);
% [numw,~] = xlsread(filename,xlRange);

% Reading MetOcean data directly from parameters
Vreq = speed;

Course=course;
% heading=Wave_Heading(legstep); %numw(4);
% period=Wave_Period(legstep); %numw(6);
% Hs=Wave_HS(legstep); %numw(5);


end

== matlab function Main_RT/Get MetOcean conditions/translate states into values 
for sea parameters ==
function [Hs_sea, Hsd_sea, Tp_sea] = weatherValues(HsSea_S, HsdSea_S, TpSea_S, leg, Hs_seaRange, Hsd_seaRange, Tp_seaRange)



Hs_sea = Hs_seaRange(HsSea_S, leg);
Hsd_sea = Hsd_seaRange(HsdSea_S, leg);
Tp_sea = Tp_seaRange(TpSea_S, leg);

end

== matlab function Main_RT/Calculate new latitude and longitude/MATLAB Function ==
function [lat_new, lon_new] = New_Lat_Lon(V_act,Course,Lat,Lon)

coder.extrinsic('nm2deg')
coder.extrinsic('reckon')
time=1; % one hour time steps

lat_new=0; %preallocate
lon_new=0; %preallocate


distance=V_act*time; %distance sailed [nm]
arc_length=nm2deg(distance); %distance sailed [deg]

[lat_new, lon_new]=reckon(Lat,Lon,arc_length,Course); %new lat and lon


end

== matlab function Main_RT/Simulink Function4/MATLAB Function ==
function [Lat1, Lon1, v_req, capacity]= SetStartAttributes(wpts,v_req_start,ship_cargo_capacity)

start=zeros(1,2);
v_req=0;

start(1,1)=wpts(1,1); %Starting Latitude
start(1,2)=wpts(1,2); %Starting Longitute

Lat1=start(1,1);
Lon1=start(1,2);

v_req=v_req_start;

capacity=ship_cargo_capacity;
end

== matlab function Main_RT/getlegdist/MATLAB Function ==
function [course,legdist] = fcn(leg,distnm_legs,course_legs)
%take in the current leg that the vessel is on, and give the distance for
%that leg, and the course
course=course_legs(leg);
legdist=distnm_legs(leg);
    
end

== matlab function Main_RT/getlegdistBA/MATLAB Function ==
function [course,legdist] = fcn(leg,distnm_legsBA,course_legsBA)
%take in the current leg that the vessel is on, and give the distance for
%that leg, and the course
course = course_legsBA(leg);
legdist = distnm_legsBA(leg);
    
end

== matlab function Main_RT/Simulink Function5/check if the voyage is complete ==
function outport = fcn(leg,legdist,dist_sailed_leg,distnm_legs)

dist=dist_sailed_leg; %the distance sailed on current leg

if leg == length(distnm_legs) && dist>=(legdist-20) %subtract to avoid errors
    outport=1; %Journey complete
else
    outport=2; %Journey not complete
end

== matlab function Main_RT/Get MetOcean conditions/translate states into values
for wind parameters1 ==
function [u10, u10d] = weatherValues_wind(leg, u10_S, u10d_S, u10_Range, u10d_Range)
                                           

u10 = u10_Range(u10_S, leg);
u10d = u10d_Range(u10d_S, leg);

end

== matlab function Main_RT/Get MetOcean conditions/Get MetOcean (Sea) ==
function [Sea_HSS, Sea_HSDS, Sea_TPS] = MC_Sea (Hs_SeS, Hsd_SeS, Tp_SeS, MC_Hs_sea, MC_Hsd_sea, MC_Tp_sea,leg,Random_Values)

persistent randnum

if isempty(randnum)
    randnum=1;
end

    
% state=0;
% P=0;
% numStates = 0;
r=0;
Sea_HSS = 0;
Sea_HSDS = 0;
Sea_TPS = 0;

%% Run through for each of the separate Markov Chains
for three_mat=1:3
    if three_mat==1
        P = MC_Hs_sea;
%         numStates = length(MC_Hs_sea(:,:,1));
        state = Hs_SeS;
        col=1;
    elseif three_mat==2
        P = MC_Hsd_sea;
%         numStates = length(MC_Hsd_sea(:,:,1));
        state = Hsd_SeS;
        col=2;
    else %three_mat==3
        P= MC_Tp_sea;
%         numStates = length(MC_Tp_sea(:,:,1));
        state = Tp_SeS;
        col=3;
    end
    
    

%% Find accumulative probability for each state, to be able to determine
%starting state

if state == 0 || state > length(P(:,:,1))
        LongRunP1=P(:,:,leg)^1000;
        PStart = zeros(length(LongRunP1),1);
        PStart (1) = LongRunP1(1,1);
            for i =2:length(LongRunP1)
                PStart (i) = PStart(i-1)+ LongRunP1(i,i);
            end

        %%  Determine starting state
        r=Random_Values(randnum,col);
        randnum=randnum+1;
        count = 1;

        if r >=1
            count = length(P(:,:,1));
        else

            while r > PStart (count)
                count = count + 1;
            end
        end

        state = count;

else
%% Find next state from previous

    cum_dist = cumsum(P(state,:,leg));
    
    iter = 0;
    r=Random_Values(randnum,col);
        randnum=randnum+1;
    temp = find(cum_dist>r);

    while isempty(temp) == 1 && iter < 100
        r=Random_Values(randnum,col);
        randnum=randnum+1;
        temp = find(cum_dist>r);
        iter = iter + 1;
    end

    if isempty(temp) == 1
        temp = state;
    end
state = temp(1);
    

end


    if three_mat==1
            Sea_HSS = state;
    elseif three_mat==2
            Sea_HSDS = state;
    else % three_mat==3
            Sea_TPS = state;
    end

end

end

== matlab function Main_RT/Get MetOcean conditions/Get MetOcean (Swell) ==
function [HS_S, HSD_S, TM_S] = MC_Swell (Wave_S, Head_S, Per_S, MC_Hs_swl, MC_Hsd_swl, MC_Tp_swl,leg,Random_Values)

persistent randnum2

if isempty(randnum2)
    randnum2=1;
end

 
% state=0;
% P=0;
% numStates = 0;
r=0;
HS_S = 0;
HSD_S = 0;
TM_S = 0;

%% Run through for each of the separate Markov Chains
for three_mat=1:3
    if three_mat==1
        P = MC_Hs_swl;
%         numStates = length(MC_Hs_swl(:,:,1));
        state = Wave_S;
        col=4;
    elseif three_mat==2
        P = MC_Hsd_swl;
%         numStates = length(MC_Hsd_swl(:,:,1));
        state = Head_S;
        col=5;
    else 
        P= MC_Tp_swl;
%         numStates = length(MC_Tp_swl(:,:,1));
        state = Per_S;
        col=6;
    end


%% Find accumulative probability for each state, to be able to determine 
%  starting state

if state == 0 || state > length(P(:,:,1))
        LongRunP1=P(:,:,leg)^1000;
        PStart = zeros(length(LongRunP1),1);
        PStart (1) = LongRunP1(1,1);
            for i =2:length(LongRunP1)
                PStart (i) = PStart(i-1)+ LongRunP1(i,i);
            end    

%%  Determine starting state
        r=Random_Values(randnum2,col);
        randnum2=randnum2+1;
        count = 1;

        if r ==1
            count = length(P(:,:,1));
        else

            while r > PStart (count)
                count = count + 1;
            end
        end
state = count;

else
%% Find next state from previous

    cum_dist = cumsum(P(state,:,leg));
    iter = 0;
    r=Random_Values(randnum2,col);
    randnum2=randnum2+1;
    temp = find(cum_dist>r);

    while isempty(temp) == 1 && iter < 100
        r=Random_Values(randnum2,col);
        randnum2=randnum2+1;
        temp = find(cum_dist>r);
        iter = iter + 1;
    end

    if isempty(temp) == 1
        temp = state;
    end

%     count = 1;
%     cum_dist = cumsum(P(state,:,leg));
% 
%     if r>=1
%     count = length(cum_dist);
% 
%     else 
%         while r > cum_dist(count)
%             count = count + 1;
%         end
%     end
% 
% % clear Sum_Check
state = temp(1); % Choose first location greater than r

end
    if three_mat==1
            HS_S = state;
    elseif three_mat==2
            HSD_S = state;
    else 
            TM_S = state;
    end


end

end

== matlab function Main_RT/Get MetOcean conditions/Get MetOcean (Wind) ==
function [u10_S, u10d_S] = MC_Wind (windVel_S, windDir_S, leg,  MC_u10, MC_u10d,Random_Values)

persistent randnum3

if isempty(randnum3)
    randnum3=1;
end
% state=0;
% P=0;
% numStates = 0;
r=0;
u10_S = 0;
u10d_S = 0;

%% Run through for each of the separate Markov Chains
for three_mat=1:2
    if three_mat==1
        P = MC_u10;
        state = windVel_S;
        col=7;
    else
        P = MC_u10d;
        state = windDir_S;
        col=8;
    end
%% Find accumulative probability for each state, to be able to determine 
%  starting state

if state == 0 || state > length(P(:,:,1))
        LongRunP1=P(:,:,leg)^1000;
        PStart = zeros(length(LongRunP1),1);
        PStart (1) = LongRunP1(1,1);
            for i =2:length(LongRunP1)
                PStart (i) = PStart(i-1)+ LongRunP1(i,i);
            end    

%%  Determine starting state
        r=Random_Values(randnum3,col);
        randnum3=randnum3+1;
        count = 1;

        if r ==1
            count = length(P(:,:,1));
        else

            while r > PStart (count)
                count = count + 1;
            end
        end
state = count;

else
%% Find next state from previous

    cum_dist = cumsum(P(state,:,leg));
    iter = 0;
    r=Random_Values(randnum3,col);
    randnum3=randnum3+1;
    temp = find(cum_dist>r);

    while isempty(temp) == 1 && iter < 100
         r=Random_Values(randnum3,col);
        randnum3=randnum3+1;
        temp = find(cum_dist>r);
        iter = iter + 1;
    end

    if isempty(temp) == 1
        temp = state;
    end

state = temp(1); % Choose first location greater than r

end
    if three_mat==1
            u10_S = state;
    else
            u10d_S = state;
    end


end

end
